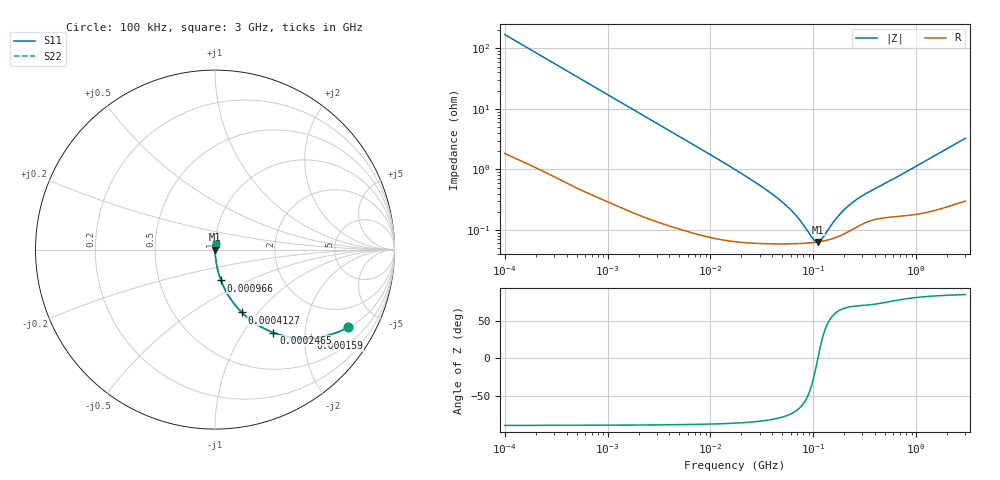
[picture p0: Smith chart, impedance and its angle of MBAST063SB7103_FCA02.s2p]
! MBAST063SB7103_FCA02  S-PARAMETER MODEL  ( Standard Model )
! Model Generated by TAIYO YUDEN Corporation (https://www.yuden.co.jp/en/)
! Version 1.0
! TAIYO YUDEN Control No. 250312
! Copyright(c) 2025 TAIYO YUDEN CO.,LTD. All Rights Reserved.
! Product Description (link to TY-COMPAS)
! https://ds.yuden.co.jp/TYCOMPAS/or/detail?pn=MBAST063SB7103KFCA02&u=M
! Products Name : Multilayer Ceramic Capacitors
! Characteristics :
!  Capacitance : 0.01 [uF] , Rated Voltage : 25 [V] , TCC : X7R
!  Case Size : 0.6 x 0.3 / 0.024 x 0.012 [mm/inch] , Thickness : 0.3 / 0.012 [mm/inch]
!  (Conditions: Temperature = 25 [degC] , DC Bias Voltage = 0 [V])
! External Node Assignments :
!  1  o---| |---o  2
! GND o---------o GND
! Frequency Range : 100kHz  -  3GHz  [ 401 STEP ]
# MHZ S RI R 50
! Freq[MHz].  S11 Real  S11 Imag  S21 Real  S21 Imag  S12 Real  S12 Imag  S22 Real  S22 Imag
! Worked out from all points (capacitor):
!   401 points, 100 kHz to 3 GHz, reference 50 ohm
!   read as one part in series: C = 9.39 nF near 105.3 kHz
!   lowest |Z| = 63.6 mohm at 110.8 MHz (marker M1)
!   series resonance near 110.6 MHz, so ESL is about 220 pH
!   S11 on the Smith chart (normalised r, x): 100 kHz: 1.04, -3.38; 159 kHz: 1.03, -2.13; 246.5 kHz: 1.02, -1.38; 412.7 kHz: 1.01, -0.83; 966 kHz: 1.01, -0.36; 3 GHz: 1.01, +0.07
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0.1  0.739 -0.4338  0.261 0.4338  0.261 0.4338  0.739 -0.4338
0.159027  0.5322 -0.493  0.4678 0.493  0.4678 0.493  0.5322 -0.493
0.246461  0.3254 -0.4621  0.6746 0.4621  0.6746 0.4621  0.3254 -0.4621
0.318916  0.2258 -0.4114  0.7742 0.4114  0.7742 0.4114  0.2258 -0.4114
0.412671  0.1501 -0.3503  0.8499 0.3503  0.8499 0.3503  0.1501 -0.3503
0.562235  0.0885 -0.2767  0.9115 0.2767  0.9115 0.2767  0.0885 -0.2767
0.965977  0.0335 -0.1718  0.9665 0.1718  0.9665 0.1718  0.0335 -0.1718
1.659646  0.0127 -0.1028  0.9873 0.1028  0.9873 0.1028  0.0127 -0.1028
3.161081  0.00434 -0.0548  0.9957 0.0548  0.9957 0.0548  0.00434 -0.0548
17.7727  0.000731 -0.00968  0.9993 0.00968  0.9993 0.00968  0.000731 -0.00968
33.85116  0.000616 -0.00474  0.9994 0.00474  0.9994 0.00474  0.000616 -0.00474
52.46276  0.000596 -0.00262  0.9994 0.00262  0.9994 0.00262  0.000596 -0.00262
71.47675  0.000599 -0.00145  0.9994 0.00145  0.9994 0.00145  0.000599 -0.00145
97.38194  0.000619 -0.00041  0.9994 0.00041  0.9994 0.00041  0.000619 -0.00041
105.21  0.000628 -0.00016  0.9994 0.00016  0.9994 0.00016  0.000628 -0.00016
110.7752  0.000636 5.99e-06  0.9994 -5.99e-06  0.9994 -5.99e-06  0.000636 5.99e-06
122.8043  0.000655 0.000339  0.9993 -0.000339  0.9993 -0.000339  0.000655 0.000339
171.6802  0.000772 0.00146  0.9992 -0.00146  0.9992 -0.00146  0.000772 0.00146
222.1509  0.000955 0.00237  0.999 -0.00237  0.999 -0.00237  0.000955 0.00237
302.6647  0.00127 0.0035  0.9987 -0.0035  0.9987 -0.0035  0.00127 0.0035
547.5153  0.00166 0.00617  0.9983 -0.00617  0.9983 -0.00617  0.00166 0.00617
3000  0.00404 0.0323  0.996 -0.0323  0.996 -0.0323  0.00404 0.0323
